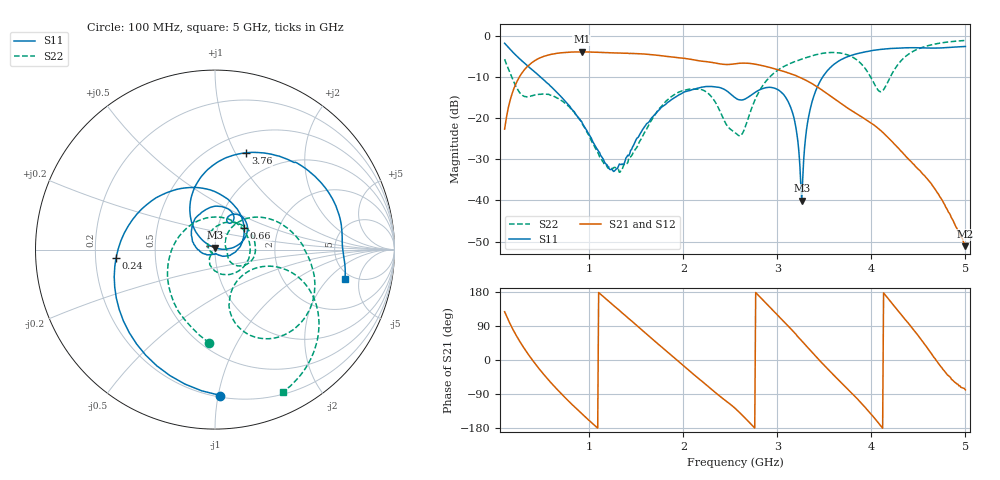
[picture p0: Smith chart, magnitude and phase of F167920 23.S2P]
!  2-Port S-parameters saved by WinCal
! VAR MeasName=S-Parameters (CALIBRATED_DATA) read from VNA (N5242A)
! VAR MeasDate=2016-11-22 9:56:18
! VAR NAME=F167920 23
! VAR FILENAME=F167920 23.S2P
! VAR DATE=2016-11-22 9:56:18
! VAR PHYS_PORTS=1,2
# Hz S DB R 50
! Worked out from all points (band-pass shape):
!   491 points, 100 MHz to 5 GHz, reference 50 ohm
!   highest |S21| = -3.88 dB at 920 MHz (marker M1); lowest = -51.1 dB at 5 GHz (marker M2)
!   |S21| within 3 dB of the highest: 370.4 MHz to 2.411 GHz (2.04 GHz wide, 147 % of centre); 2.522 GHz to 2.764 GHz (242.3 MHz wide, 9.17 % of centre)
!   lowest |S11| = -40.1 dB at 3.26 GHz (marker M3), VSWR 1.02, Z = 50.1 + j0.987 ohm
!   |S11| at or under -10 dB: 481.2 MHz to 3.482 GHz (3.001 GHz wide, 151 % of centre)
!   |S22| runs from -33.2 to -1.1 dB; largest |S21 - S12| = 0.0011
!   S11 on the Smith chart (normalised r, x): 100 MHz: 0.21, -1.02; 240 MHz: 0.29, -0.04; 660 MHz: 1.34, +0.34; 3.76 GHz: 0.69, +1.10; 5 GHz: 4.36, -3.19
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1e8  -1.79 -87.9  -22.67 127.4  -22.67 127.6  -5.66 -93.5
1.7e8  -3.55 -136.0  -14.73 89.6  -14.73 89.6  -9.67 -141.7
2.4e8  -5.15 -175.4  -10.71 57.8  -10.71 57.8  -13.08 166.8
4.4e8  -9.15 101.3  -5.77 -14.6  -5.76 -14.6  -14.27 35.4
6.6e8  -13.85 37.2  -4.23 -78.0  -4.23 -78.0  -15.12 -44.3
9.2e8  -20.85 -20.8  -3.88 -141.5  -3.87 -141.5  -21.06 -109.3
1.21e9  -32.25 -73.1  -4.10 154.2  -4.10 154.2  -31.87 -122.2
1.33e9  -31.24 -107.8  -4.15 128.6  -4.14 128.6  -33.05 -141.4
1.74e9  -18.07 163.3  -4.76 40.5  -4.76 40.5  -17.83 87.5
1.96e9  -14.26 128.5  -5.34 -6.0  -5.34 -6.0  -13.60 37.2
2.2e9  -12.47 94.6  -6.16 -56.4  -6.16 -56.5  -13.09 -9.6
2.55e9  -15.01 58.2  -6.78 -127.2  -6.79 -127.2  -23.53 -6.0
2.78e9  -13.51 65.9  -6.95 175.4  -6.95 175.4  -14.69 51.1
3.07e9  -14.35 24.6  -8.66 101.7  -8.66 101.6  -7.44 15.7
3.18e9  -20.23 5.7  -9.49 72.7  -9.49 72.6  -6.30 3.9
3.26e9  -40.06 82.6  -10.31 50.3  -10.29 50.2  -5.64 -4.6
3.37e9  -15.97 135.5  -11.61 20.2  -11.61 20.1  -4.82 -15.3
3.76e9  -4.95 72.5  -17.73 -79.4  -17.76 -79.4  -4.73 -58.9
4.09e9  -3.32 39.6  -22.84 -170.6  -22.88 -170.5  -13.53 -50.6
4.19e9  -3.10 31.5  -24.99 158.5  -25.02 158.6  -10.51 -18.1
4.49e9  -2.89 10.7  -32.22 67.0  -32.19 67.0  -3.25 -32.9
5e9  -2.58 -12.8  -51.12 -78.8  -50.77 -77.3  -1.12 -64.4
